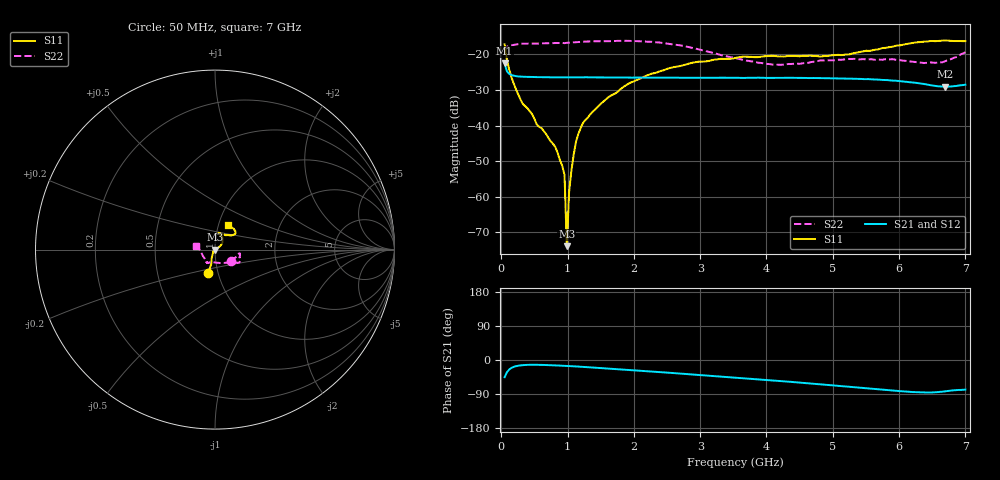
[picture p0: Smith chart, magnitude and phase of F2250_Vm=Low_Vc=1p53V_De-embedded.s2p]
! Integrated Device Technology
! Corporate Headquarters
! 6024 Silver Creek Valley Road
! San Jose, CA 95138  USA
! Phone:  1-408-284-8200
! Toll Free:  1-800-223-1366
! Webpage:  http://www.idt.com/
! Timing and RF Division
! 515 Groton Road, Suite 102
! Westford, MA 01886-6024
! Device:  F2250
! Description: Voltage Variable RF Attenuator
! Frequency:  50.0 -  6000.00 MHz
! Package:  3x3 mm Thin QFN Plastic Package: 16 pin
! Ports:  2 RF, 3 DC
!  Pin  1  = GND
!  Pin  2  = NC
!  Pin  3  = RF1  = Port 1
!  Pin  4  = NC
!  Pin  5  = GND
!  Pin  6  = GND
!  Pin  7  = GND
!  Pin  8  = GND
!  Pin  9  = NC
!  Pin 10  = RF2  = Port 2
!  Pin 11  = NC
!  Pin 12  = GND
!  Pin 13  = GND
!  Pin 14  = VCNTRL
!  Pin 15  = VDD
!  Pin 16  = VMODE
! Vcntrl:  1.530 Volts
! Vmode:  +0.000 Volts
! Vdd:  +3.30  Volts
! Current:  1.191 mA
! Data:  The device was measured on a the F2250 evaluation board which has
!  individual transmission lines to the RF pins.  Data was collected
!  using a calibrated network analyzer.  The evaluation board was
!  de-embedded using a TRL calibration technique.
!  The reference plane is the edge of the package pin.
! Misc:  SN 10
!  Action Tracker AT0258
! Date Measured:  2014-11-26
! Date:  2015-10-15  MJV
! Note:
!  Integrated Device Technology supplies this data as a sample of measured
!  data at the package pin for this product.  Your particular data for this
!  product may vary.
!  Data was taken at 25 degrees C.
!  Integrated Device Technology reserves the right to change this data at anytime.
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# GHz S dB R 50
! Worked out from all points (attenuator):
!   201 points, 50 MHz to 7 GHz, reference 50 ohm
!   highest |S21| = -22.58 dB at 50 MHz (marker M1); lowest = -29.1 dB at 6.687 GHz (marker M2)
!   lowest |S11| = -73.9 dB at 988.2 MHz (marker M3), VSWR 1.00, Z = 50 + j0.0106 ohm
!   |S11| at or under -10 dB: start of sweep to end of sweep
!   |S22| runs from -23.0 to -16.2 dB; largest |S21 - S12| = 0.00022
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0.05  -17.20 -106.6  -22.58 -45.4  -22.58 -45.4  -19.34 -36.1
0.1195  -24.34 -108.1  -25.50 -25.1  -25.50 -25.1  -17.59 -12.0
0.29325  -32.83 -119.2  -26.27 -14.1  -26.27 -14.1  -17.04 -9.3
0.5365  -39.73 -142.8  -26.42 -12.7  -26.39 -12.7  -17.01 -10.9
0.8145  -46.00 179.8  -26.47 -14.2  -26.44 -14.2  -16.87 -15.6
0.91875  -51.27 153.1  -26.46 -15.1  -26.46 -15.1  -16.80 -17.6
0.9535  -53.84 -175.4  -26.46 -15.4  -26.45 -15.4  -16.88 -17.8
0.98825  -73.85 148.6  -26.46 -15.7  -26.48 -15.7  -16.79 -18.2
1.023  -58.61 25.5  -26.49 -16.0  -26.48 -16.0  -16.75 -18.3
1.05775  -52.58 28.2  -26.50 -16.3  -26.47 -16.3  -16.73 -18.7
1.12725  -44.49 25.1  -26.48 -17.0  -26.46 -17.0  -16.61 -19.9
1.2315  -39.30 25.0  -26.47 -18.1  -26.44 -18.1  -16.47 -21.7
1.5095  -33.74 30.3  -26.49 -21.4  -26.49 -21.4  -16.34 -23.9
1.857  -28.96 34.7  -26.52 -25.5  -26.51 -25.5  -16.22 -27.0
2.37825  -24.86 43.6  -26.57 -31.8  -26.57 -31.8  -16.68 -30.5
2.93425  -22.18 57.5  -26.57 -38.8  -26.56 -38.8  -18.42 -37.4
3.525  -21.06 70.8  -26.61 -46.4  -26.60 -46.4  -21.07 -58.2
4.11575  -20.44 78.6  -26.63 -54.2  -26.62 -54.2  -22.92 -88.2
4.7065  -20.47 71.4  -26.66 -62.6  -26.64 -62.7  -22.10 -112.3
5.85325  -17.99 39.5  -27.31 -79.8  -27.29 -79.9  -21.44 -123.6
6.68725  -16.12 48.2  -29.13 -82.8  -29.10 -82.8  -22.00 -172.2
7  -16.31 62.8  -28.53 -78.2  -28.49 -78.3  -19.43 168.0
